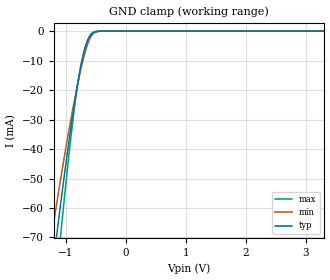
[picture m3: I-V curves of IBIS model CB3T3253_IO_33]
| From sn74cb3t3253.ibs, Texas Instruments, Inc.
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[Model]   CB3T3253_IO_33
Model_type  Terminator
| variable   typ   min   max
C_comp   3.99pF   3.07pF   5.16pF
| C_tri-state   3.99pF   3.07pF   5.16pF
[Temperature Range]   40   100   -40
| Ambient temperature   25   85   -40
[Voltage range]   3.3   3   3.6
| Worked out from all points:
|   GND clamp passes 1 mA (typ) near -0.56 V on its own axis
[GND Clamp]
| CB3T3253_IO_33
|   Voltage   I(typ)   I(min)   I(max)
-5.5V     -1.008A    -841.1mA   -1.184A
-1.24V    -84.16mA   -70.17mA   -102.1mA
-1.195V   -76.47mA   -64.15mA   -92.27mA
-1.15V    -68.95mA   -58.26mA   -82.61mA
-1.09V    -59.17mA   -50.61mA   -70.01mA
-1.07V    -55.99mA   -48.11mA   -65.89mA
-890mV    -29.27mA   -27.07mA   -31.52mA
-790mV    -16.49mA   -16.78mA   -16.36mA
-675mV    -5.462mA   -6.985mA   -5.356mA
-550mV    -740.6uA   -1.02mA    -478.1uA
-325mV    -2.166uA   -4.071uA   -187.7nA
3.3V      246.4pA    10.98nA    81.93pA
